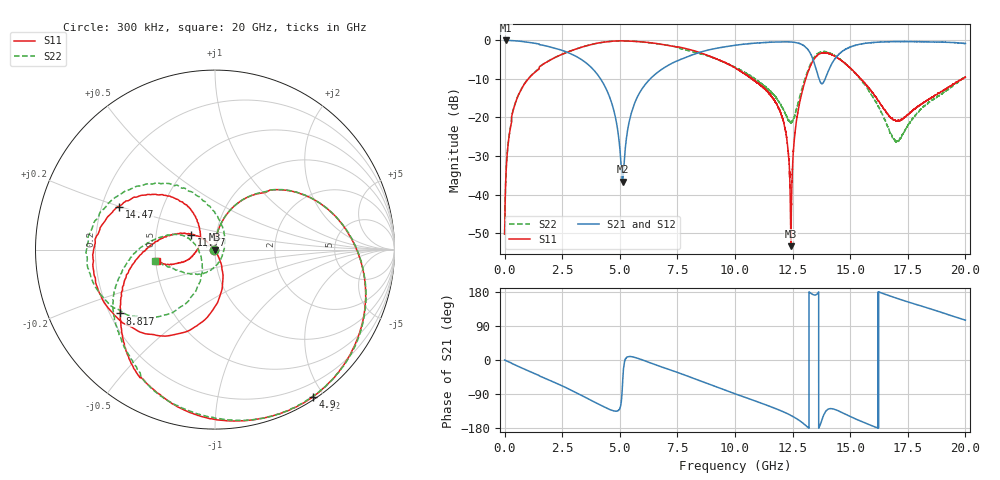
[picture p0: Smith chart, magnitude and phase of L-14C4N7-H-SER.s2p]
!{L-14C4N7}
!Johanson Technology Inc.
!www.johansontechnology.com
!Test Board Conditions:
!Substrate Type  RO4350B
!Substrate Thickness  20 mil
!Substrate Dk  3.66
!TL Type: GCPW
!TL Trace Width  36 mil
!TL Gap  12 mil
!Electrode orientation  Horizontal
!DUT TOPOLOGY	SERIES
!Mounting Pad LxW  26x36 mil
! Created Sun Jun 20 12:57:51 2021
# hz S ma R 50
! 2 Port Network Data from SP1.SP block
! freq  magS11  angS11  magS21  angS21  magS12  angS12  magS22  angS22
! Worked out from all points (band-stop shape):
!   20001 points, 300 kHz to 20 GHz, reference 50 ohm
!   highest |S21| = -0.02 dB at 72.3 MHz (marker M1); lowest = -36.6 dB at 5.118 GHz (marker M2)
!   |S21| within 3 dB of the highest: 8.517 GHz to 13.24 GHz (4.721 GHz wide, 43.4 % of centre); 14.62 GHz to end of sweep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
!   lowest |S11| = -53.4 dB at 12.42 GHz (marker M3), VSWR 1.00, Z = 49.8 - j0.0157 ohm
!   |S11| at or under -10 dB: start of sweep to 1.028 GHz; 10.74 GHz to 13.07 GHz (2.327 GHz wide, 19.5 % of centre); 15.47 GHz to 19.87 GHz (4.406 GHz wide, 24.9 % of centre)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
!   |S22| runs from -50.5 to -0.1 dB; largest |S21 - S12| = 0.013
!   S11 on the Smith chart (normalised r, x): 300 kHz: 0.99, +0.00; 4.9 GHz: 0.03, -1.87; 8.817 GHz: 0.24, -0.29; 11.77 GHz: 0.76, +0.13; 14.47 GHz: 0.27, +0.20; 20 GHz: 0.51, -0.07
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300000  0.003065 176.1  0.998 -0.0  0.9955 -0.0  0.002985 -177.7
7.23e7  0.02193 93.3  0.9982 -2.0  0.9974 -2.0  0.02208 92.8
3.093e8  0.1036 81.2  0.9942 -8.9  0.9939 -8.9  0.1045 81.1
7.583e8  0.2421 68.2  0.9677 -21.4  0.9681 -21.3  0.2444 68.3
3.3343e9  0.8147 -4.5  0.5645 -93.2  0.5655 -93.1  0.8141 -4.0
4.3613e9  0.9551 -38.6  0.2503 -125.2  0.2511 -125.3  0.9559 -37.7
4.9003e9  0.9851 -56.2  0.07117 -134.3  0.07117 -134.1  0.9816 -55.1
5.1183e9  0.9855 -62.9  0.01473 -63.2  0.01482 -63.3  0.9849 -61.8
5.6203e9  0.973 -77.0  0.1469 7.2  0.147 7.3  0.9732 -75.8
6.6673e9  0.9047 -102.4  0.3906 -15.2  0.3911 -14.8  0.8992 -102.3
8.8173e9  0.6369 -146.0  0.7477 -62.4  0.7466 -62.5  0.632 -154.1
1.00003e10  0.441 -172.8  0.8631 -89.1  0.8657 -89.1  0.4489 -177.3
1.17723e10  0.1559 147.8  0.9526 -128.5  0.9538 -128.6  0.1814 155.9
1.21713e10  0.07192 136.5  0.9594 -138.7  0.959 -138.7  0.1133 165.7
1.24213e10  0.002138 -175.8  0.9541 -146.2  0.9567 -146.2  0.08576 -161.8
1.27413e10  0.1221 -70.7  0.9207 -157.6  0.9251 -157.5  0.1553 -118.5
1.33343e10  0.5098 -113.3  0.6196 174.3  0.6223 174.0  0.5352 -134.4
1.37813e10  0.6859 -157.8  0.2742 -156.6  0.2734 -157.6  0.7129 -171.2
1.44683e10  0.5871 155.9  0.642 -133.8  0.6414 -134.0  0.5952 146.7
1.66673e10  0.1068 138.8  0.9614 170.2  0.9624 170.5  0.07259 40.4
1.70603e10  0.09098 164.0  0.9662 162.1  0.9669 162.3  0.04955 -21.8
2e10  0.3317 -168.7  0.9111 105.1  0.8996 104.8  0.3426 -169.8
